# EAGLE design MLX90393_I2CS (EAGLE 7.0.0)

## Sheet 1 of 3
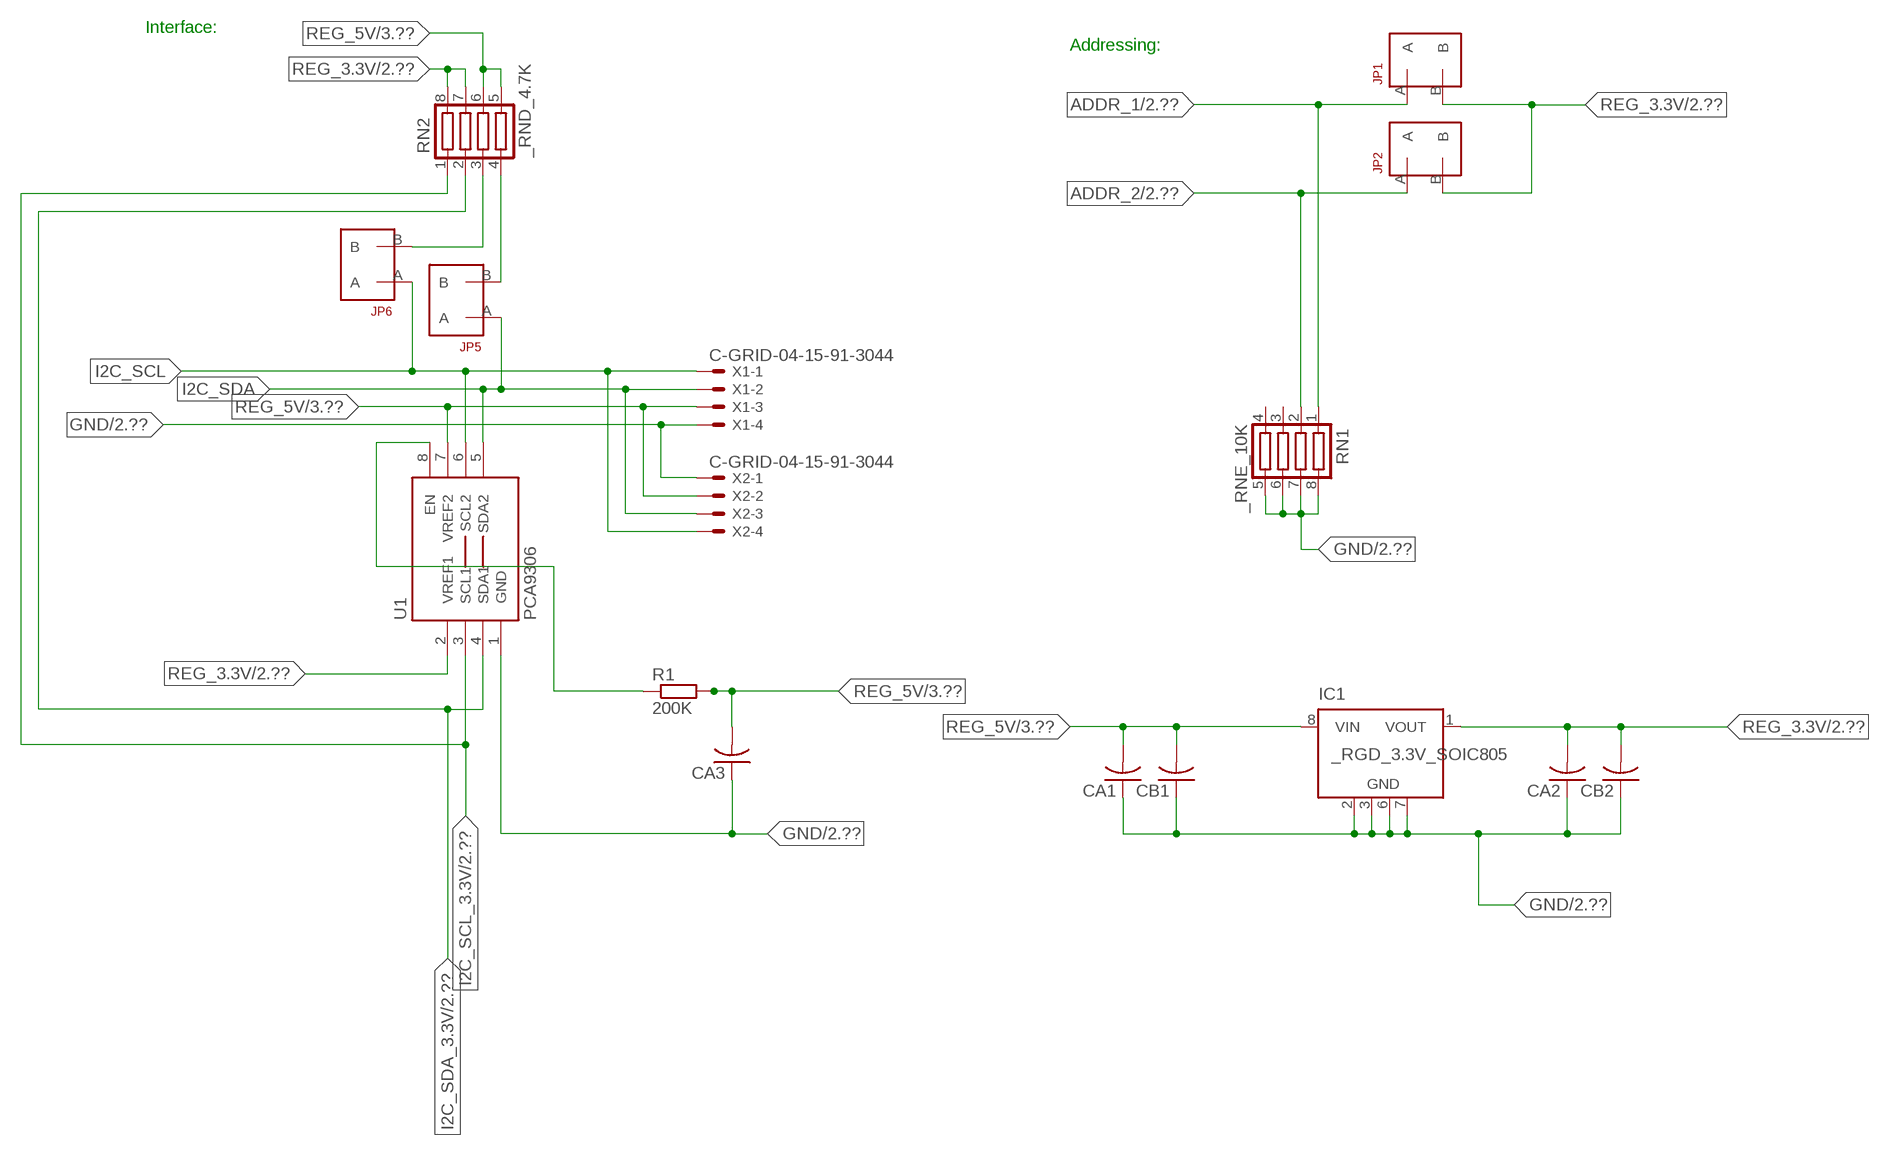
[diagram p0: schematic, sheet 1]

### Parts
CA1  CC1206KRX7R9BB104  [.1UF]
CA2  CC1206KRX7R9BB104  [.1UF]
CA3  CC1206KRX7R9BB104  [.1UF]
CB1  TMK316F106ZL-TC1206K  [TMK316F106ZL-T]
CB2  TMK316F106ZL-TC1206K  [TMK316F106ZL-T]
IC1  _RGD_3.3V_SOIC805  [_RGC_3.3V_SOIC8]
JP1  JUMPER_1X2_2MM  [JUMPER_1X2_2MM]
JP2  JUMPER_1X2_2MM  [JUMPER_1X2_2MM]
JP5  JUMPER_1X2_2MM  [JUMPER_1X2_2MM]
JP6  JUMPER_1X2_2MM  [JUMPER_1X2_2MM]
R1  200K  RESISTOR_SMT-0603  [R603]
RN1  _RNE_10K  [RNE]
RN2  _RND_4.7K  [RND]
U1  PCA9306  PCA9306_NCD  [PSOP-8]
X1  C-GRID-04-15-91-3044  [15-91-04]
X2  C-GRID-04-15-91-3044  [15-91-04]

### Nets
ADDR_1: JP1.A RN1.1 ; also sheet 2
ADDR_2: JP2.A RN1.2 ; also sheet 2
GND: CA1.1 CA2.1 CA3.1 CB1.1 CB2.1 IC1.2(GND) IC1.3(GND) IC1.6(GND) IC1.7(GND) RN1.5 RN1.6 RN1.7 RN1.8 U1.1(GND) X1.4 X2.1 ; also sheet 2,3
I2C_SCL: JP6.A U1.6(SCL2) X1.1 X2.4
I2C_SCL_3.3V: RN2.1 U1.3(SCL1) ; also sheet 2
I2C_SDA: JP5.A U1.5(SDA2) X1.2 X2.3
I2C_SDA_3.3V: RN2.2 U1.4(SDA1) ; also sheet 2
N$1: JP6.B RN2.3
N$2: JP5.B RN2.4
N$3: R1.1 U1.8(EN)
REG_3.3V: CA2.2 CB2.2 IC1.1(VOUT) JP1.B JP2.B RN2.7 RN2.8 U1.2(VREF1) ; also sheet 2
REG_5V: CA1.2 CA3.2 CB1.2 IC1.8(VIN) R1.2 RN2.5 RN2.6 U1.7(VREF2) X1.3 X2.2 ; also sheet 3
Unconnected: IC1.4(NC) IC1.5(NC) RN1.3 RN1.4

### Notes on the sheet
- Interface:
- Addressing:

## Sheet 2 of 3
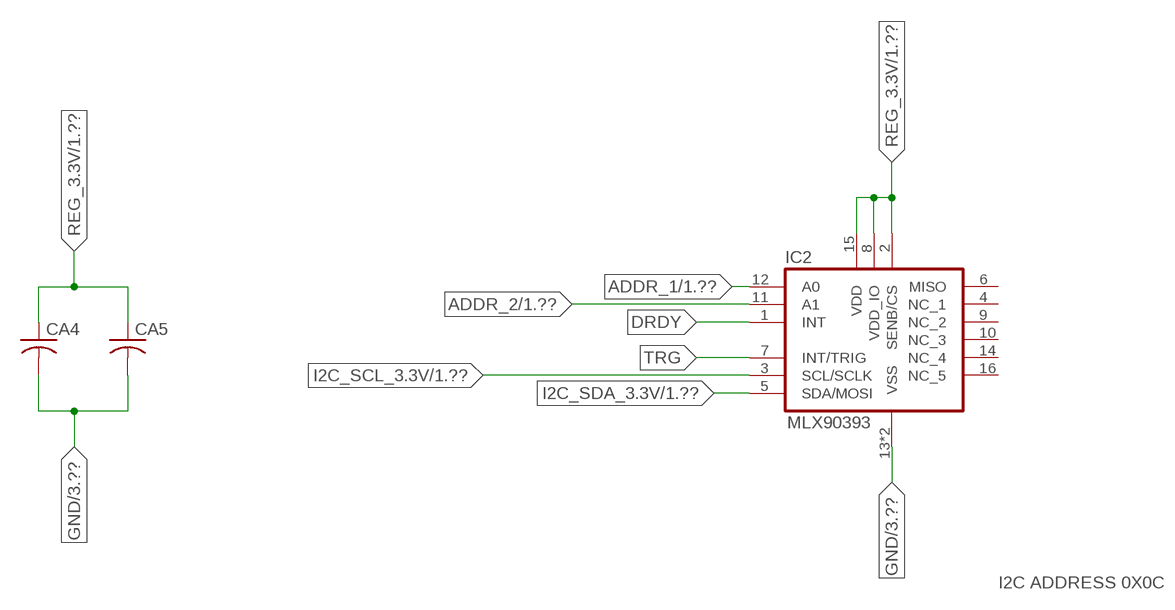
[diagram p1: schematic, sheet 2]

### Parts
CA4  CC1206KRX7R9BB104C1206K  [CC1206KRX7R9BB104]
CA5  CC1206KRX7R9BB104C1206K  [CC1206KRX7R9BB104]
IC2  MLX90393  [MLX90393]

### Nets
ADDR_1: IC2.12(A0) ; also sheet 1
ADDR_2: IC2.11(A1) ; also sheet 1
DRDY: IC2.1(INT)
GND: CA4.2 CA5.2 IC2.13(VSS) IC2.TH(VSS) ; also sheet 1,3
I2C_SCL_3.3V: IC2.3(SCL/SCLK) ; also sheet 1
I2C_SDA_3.3V: IC2.5(SDA/MOSI) ; also sheet 1
REG_3.3V: CA4.1 CA5.1 IC2.2(SENB/CS) IC2.8(VDD_IO) IC2.15(VDD) ; also sheet 1
TRG: IC2.7(INT/TRIG)
Unconnected: IC2.4(NC_1) IC2.6(MISO) IC2.9(NC_2) IC2.10(NC_3) IC2.14(NC_4) IC2.16(NC_5)

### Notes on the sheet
- I2C ADDRESS 0X0C

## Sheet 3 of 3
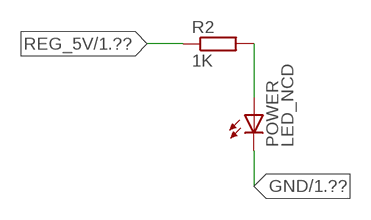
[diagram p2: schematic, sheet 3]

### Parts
POWER  LED_NCD  [CHIPLED_0603]
R2  1K  RESISTOR_SMT-0402  [R402]

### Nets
GND: POWER.C ; also sheet 1,2
N$4: POWER.A R2.2
REG_5V: R2.1 ; also sheet 1

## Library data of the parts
CA1-CA5 = NCD_ULTIMATE_LIBRARY:CC1206KRX7R9BB104: Capacitor CA .1uF 50V SMT C1206K CC1206KRX7R9BB104
CB1 CB2 = NCD_ULTIMATE_LIBRARY:TMK316F106ZL-T: Capacitor CB 10uF SMT 1206 TMK316F106ZL-T
IC1 = NCD_ULTIMATE_LIBRARY:_RGD_3.3V_SOIC8: Regulator Linear 3.3V Chip Positive VOLTAGE REGULATOR Digikey 497-1199-2-ND/L78L33ACD13TR
IC2 = NCD_ULTIMATE_AMAN:MLX90393
JP1 JP2 JP5 JP6 = NCD_ULTIMATE_CONNECTORS:JUMPER_1X2_2MM
POWER = NCD_ULTIMATE_LIBRARY:LED_NCD: LED Digikey 754-1132-2-ND/APT2012SRCPRV
R1 R2 = NCD_ULTIMATE_LIBRARY:RESISTOR_SMT: NCD Resistor
RN1 = NCD_ULTIMATE_LIBRARY:_RNE_10K: Resistor Array RNE SMT 10K x 4 Single Resistor Source: http://www.ctscorp.com/components/Datasheets/CTSChipArrayDs.pdf Digikey 742C083103JPTR-ND/742C083103JP; OC_FARNELL: unknown; OC_NEWARK: unknown
RN2 = NCD_ULTIMATE_LIBRARY:_RND_4.7K: Resistor Array RND SMT 4.7K x 4 Single Resistor Source: http://www.ctscorp.com/components/Datasheets/CTSChipArrayDs.pdf Digikey 742C083472JPTR-ND/742C083472JP; OC_FARNELL: unknown; OC_NEWARK: unknown
U1 = NCD_ULTIMATE_LIBRARY:PCA9306_NCD: NCD Bidirectional I2C level shifter. NOT compatible with all available part number pinout schemes- DOUBLE CHECK!!!; PROD_ID: IC-10023
X1 X2 = NCD_ULTIMATE_CONNECTORS:C-GRID-04: CONNECTOR 4-Pos I2C wire to board 2.54 mm (0.100") pitch header Digikey WM1342-ND/0015912045; OC_FARNELL: unknown; OC_NEWARK: unknown

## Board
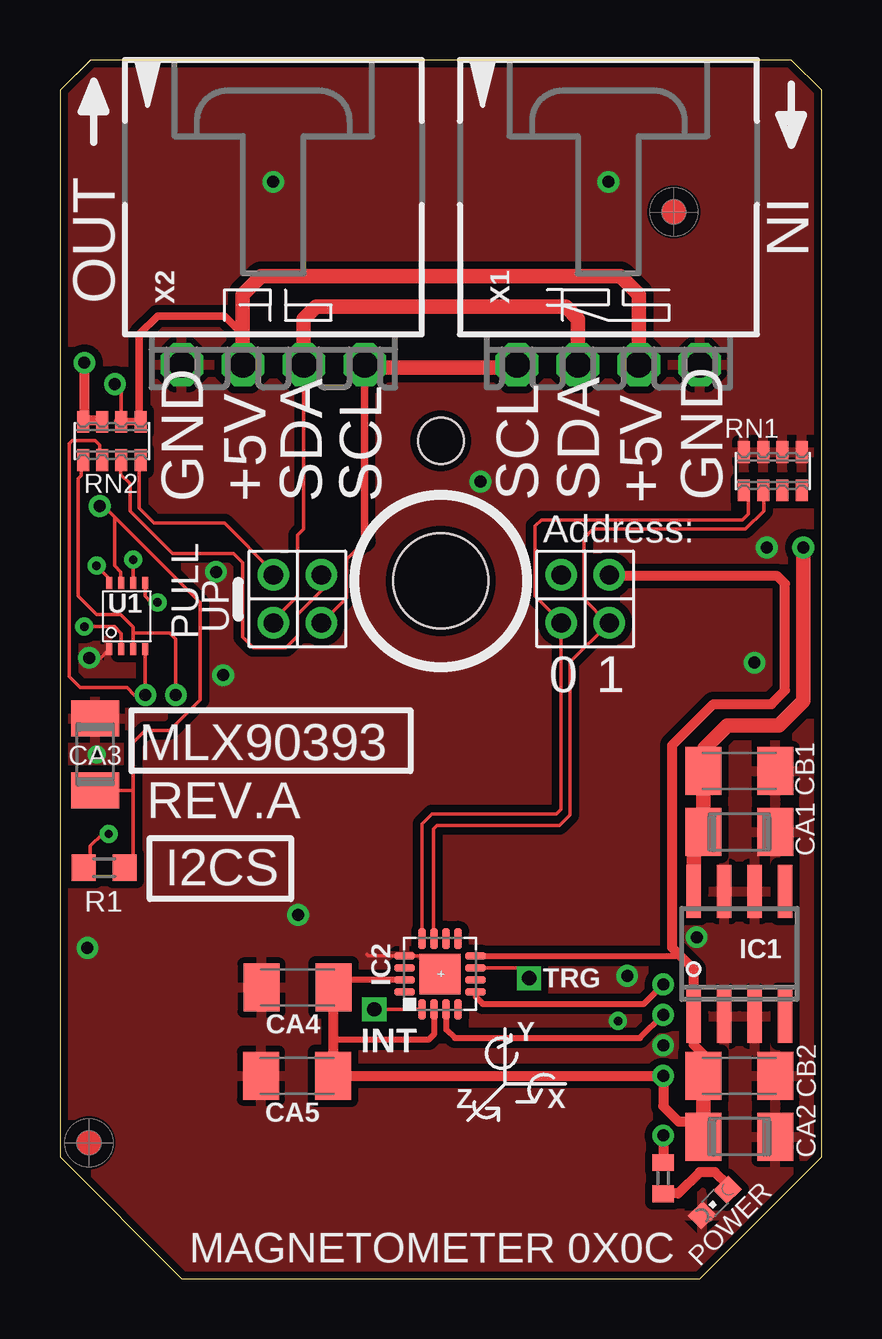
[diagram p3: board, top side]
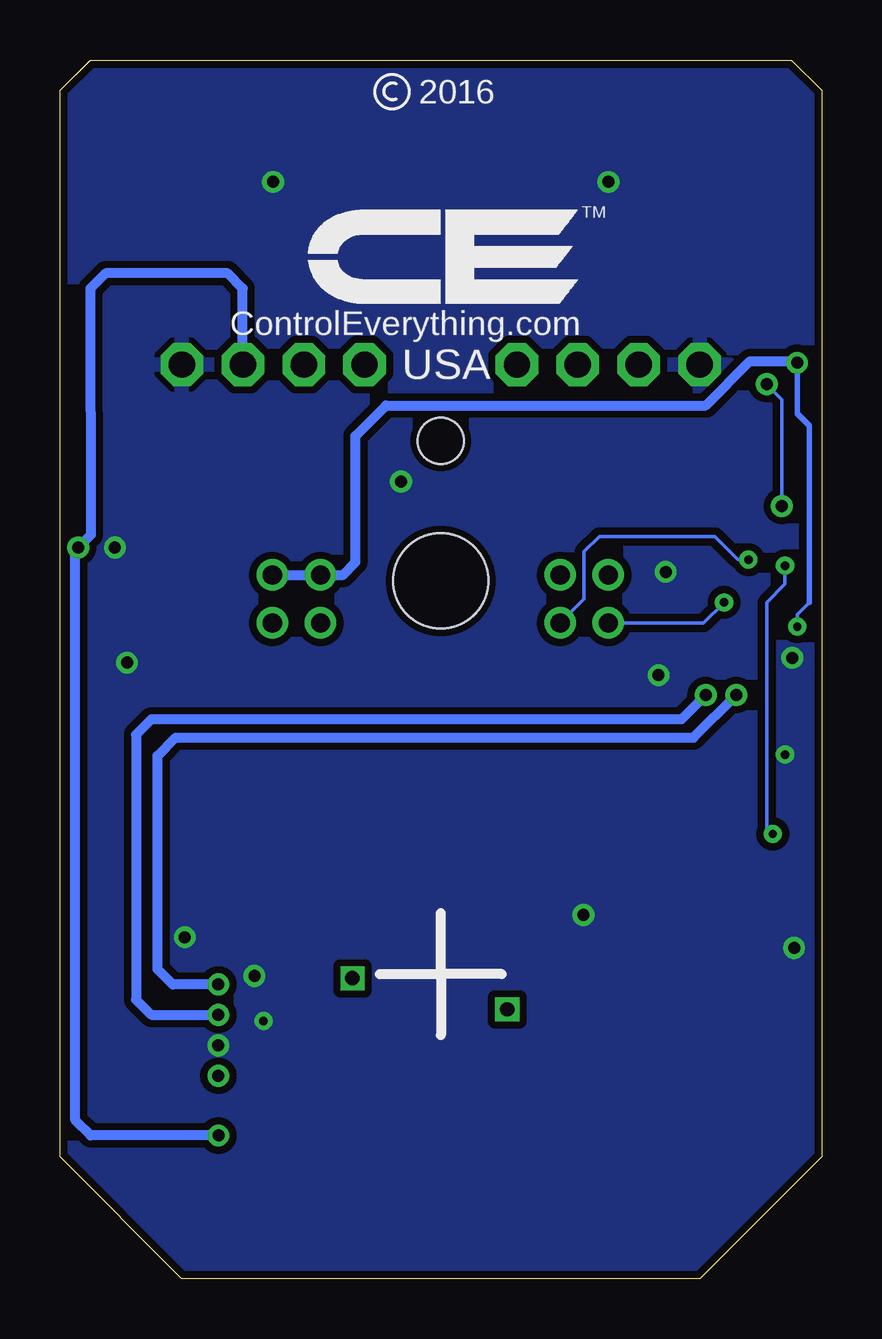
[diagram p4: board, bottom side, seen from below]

Size 31.75 x 50.8 mm. Coordinates in mm from the lower left corner, seen from the top.
Outline: 48 segments
Copper layers (1*16): Top 0.035mm / dielectric 1.5mm / Bottom 0.035mm
Design rules "default": minimum track width 5mil, minimum drill 24mil, track to track 5mil, track to pad 5mil, pad to pad 5mil, via to via 5mil, smd to smd 5mil, copper to edge 10mil, drill to drill 8mil, minimum pad ring 10mil, minimum via ring 8mil, stop-mask expansion 2mil, vias tented up to drill 0mil, thermal gap 10mil
Holes 3.96 mm at 15.88,29.08
Holes 1.91 mm at 15.88,34.93

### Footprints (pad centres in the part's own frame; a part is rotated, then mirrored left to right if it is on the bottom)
.1UF = smd 1.5 x 2: 1 -1.5,0; 2 1.5,0
CC1206KRX7R9BB104 = smd 1.5 x 2: 1 -1.5,0; 2 1.5,0
TMK316F106ZL-T = smd 1.5 x 2: 1 -1.5,0; 2 1.5,0
_RGC_3.3V_SOIC8 = smd 0.6 x 2.2: 1 -1.905,-2.6; 2 -0.635,-2.6; 3 0.635,-2.6; 4 1.905,-2.6; 5 1.905,2.6; 6 0.635,2.6; 7 -0.635,2.6; 8 -1.905,2.6
MLX90393 = smd 0.85 x 0.3: 1 -1.475,0.75; 2 -1.475,0.25; 3 -1.475,-0.25; 4 -1.475,-0.75; 9 1.475,-0.75; 10 1.475,-0.25; 11 1.475,0.25; 12 1.475,0.75 | smd 0.3 x 0.85: 5 -0.75,-1.475; 6 -0.25,-1.475; 7 0.25,-1.475; 8 0.75,-1.475; 13 0.75,1.475; 14 0.25,1.475; 15 -0.25,1.475; 16 -0.75,1.475 | smd 1.7 x 1.7: TH 0,0
JUMPER_1X2_2MM = drill 0.8: A 0,2; B 0,0
CHIPLED_0603 = smd 0.8 x 0.876: A 0,-0.75; C 0,0.75
R603 = smd 1 x 1.1: 1 -0.85,0; 2 0.85,0
R402 = smd 0.7 x 0.9: 1 -0.65,0; 2 0.65,0
RNE = smd 0.5 x 0.9: 1 -1.2,-0.8; 2 -0.4,-0.8; 3 0.4,-0.8; 4 1.2,-0.8; 5 1.2,0.8; 6 0.4,0.8; 7 -0.4,0.8; 8 -1.2,0.8
RND = smd 0.5 x 0.9: 1 -1.2,-0.8; 2 -0.4,-0.8; 3 0.4,-0.8; 4 1.2,-0.8; 5 1.2,0.8; 6 0.4,0.8; 7 -0.4,0.8; 8 -1.2,0.8
PSOP-8 = smd 0.25 x 0.5: 1 -0.73,-1.37; 2 -0.23,-1.37; 3 0.27,-1.37; 4 0.77,-1.37; 5 0.77,1.38; 6 0.27,1.38; 7 -0.23,1.38; 8 -0.73,1.38
15-91-04 = drill 1.1 pad 1.778 octagon: 1 -3.81,-7.62; 2 -1.27,-7.62; 3 1.27,-7.62; 4 3.81,-7.62

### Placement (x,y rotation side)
CA1  28.32,18.62 180 top
CA2  28.32,5.92 180 top
CA3  1.46,21.86 270 top
CA4  9.91,12.14 180 top
CA5  9.88,8.46 180 top
CB1  28.32,21.16 180 top
CB2  28.32,8.46 180 top
IC1  28.32,13.54 0 top
IC2  15.85,12.7 90 top
JP1  20.89,29.34 180 top
JP2  22.9,29.34 180 top
JP5  8.89,29.34 180 top
JP6  10.9,29.34 180 top
POWER  27.3,3.18 135 top
R1  1.84,17.13 0 top
R2  25.15,4.19 270 top
RN1  29.72,33.66 0 top
RN2  2.16,34.93 0 top
U1  2.79,27.61 0 top
U$5  [VISION_REF10]  1.21,5.66 90 top
U$28  [VISION_REF10]  25.59,44.46 90 top
X1  22.86,45.72 0 top
X2  8.89,45.72 0 top

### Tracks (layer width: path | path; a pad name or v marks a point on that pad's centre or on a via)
ADDR_1
  Top 0.152: RN1.1 28.7,32.78 28.7,31.88 28.45,31.62 20.07,31.62 19.81,31.37 19.81,28.45 20.89,27.37 JP1.A 20.88,27.32 20.88,19.56 20.7,19.38 15.52,19.38 15.1,18.96 IC2.12
ADDR_2
  Top 0.152: RN1.2 29.34,32.59 29.34,32 28.57,31.24 22.23,31.24 21.84,30.86 21.84,28.32 22.83,27.34 JP2.A 21.26,25.7 21.26,19.33 20.83,18.9 15.72,18.9 15.57,18.75 15.57,14.5 15.6,14.47 IC2.11
DRDY  (via drill 0.6)
  Top 0.152: IC2.1 v13.11,11.23
GND  (via drill 0.35, 0.5)
  Top 0.152: CA3.1 1.52,23.42 1.52,23.62 | U1.1 1.7,25.88 v1.22,25.88 | IC2.TH 15.1,13.45 IC2.13 12.86,13.45 12.8,13.51
  other vias: 8.89,45.72 22.86,45.72 25.15,9.73 6.8,25.16 17.53,33.22 26.55,14.24 1.15,13.79 6.5,29.46 1.52,21.84 23.65,12.62 23.27,10.74 29.46,30.48 28.96,25.68 9.93,15.16
  pour Top (isolate 0.305): -1.27,0 -1.27,50.8 33.02,50.8 33.02,0
  pour Bottom (isolate 0.305): -5.08,0 -5.08,50.8 35.56,50.8 35.56,0
I2C_SCL  (via drill 0.35)
  Top 0.152: 12.7,30.73 11.94,29.97 11.94,28.38 JP6.A | v3.05,29.97 3.06,29.96 U1.6
  Top 0.305: 12.7,30.73 X2.4
  Top 0.406: X2.4 12.7,37.97 | 19.05,37.97 X1.1
  Top 0.61: 12.7,37.97 19.05,37.97
  Bottom 0.152: JP6.A 9.91,28.33 9.91,30.3 9.27,30.94 4.45,30.94 3.48,29.97 v3.05,29.97
I2C_SCL_3.3V  (via drill 0.5)
  Top 0.152: RN2.1 0.89,34.07 0.89,33.48 0.77,33.35 0.77,29.1 0.76,29.09 0.76,28.45 1.52,27.69 2.54,27.69 3.06,27.17 3.06,26.92 | 3.06,26.92 U1.3 | v4.83,24.33 v4.83,24.34 4.83,26.67 4.57,26.92 3.06,26.92
  Top 0.254: IC2.3 16.1,10.39 16.46,10.03 24.18,10.03 v25.15,11
  Bottom 0.406: v4.83,24.33 5.84,23.32 27.94,23.32 28.58,22.68 28.58,11.63 27.94,11 v25.15,11
I2C_SDA  (via drill 0.35)
  Top 0.152: JP5.A 8.89,27.44 9.91,28.45 9.91,30.99 10.16,31.24 10.16,34.92 X2.3 | U1.5 3.56,28.45 3.81,28.19 v4.06,28.19
  Top 0.61: X2.3 10.16,40.01 10.67,40.51 21.09,40.51 21.59,40.01 X1.2
  Bottom 0.152: v4.06,28.19 4.92,27.34 JP5.A
I2C_SDA_3.3V  (via drill 0.5)
  Top 0.152: RN2.2 1.65,34.14 1.65,34.75 1.46,34.94 0.51,34.94 0.38,34.81 0.38,26.37 0.38,26.36 0.38,25.1 0.84,24.64 2.79,24.64 3.1,24.33 v3.56,24.33 v3.56,24.34 U1.4
  Top 0.254: IC2.5 17.32,11.76 17.63,11.46 24.34,11.46 v25.15,12.27
  Bottom 0.406: v25.15,12.27 27.05,12.27 27.69,12.9 27.69,21.79 26.93,22.56 5.34,22.56 v3.56,24.33
N$1
  Top 0.152: JP6.B 10.92,29.31 10.92,28.7 9.91,27.69 9.91,26.8 9.42,26.31 8.06,26.31 7.62,26.75 7.62,29.84 7.24,30.23 4.7,30.23 2.92,32 2.92,33.15 2.54,33.53 2.54,34.1 RN2.3
  Top 0.305: 2.54,34.02 RN2.3
N$2
  Top 0.152: JP5.B 8.89,29.46 6.86,31.5 3.94,31.5 3.3,32.13 3.3,34.07 RN2.4
  Top 0.305: 3.37,33.88 RN2.4
N$3  (via drill 0.35)
  Top 0.152: R1.1 1.27,17.41 1.27,18.03 1.78,18.54 v2.03,18.54 | v1.52,29.72 2.06,29.18 U1.8
  Bottom 0.152: v2.03,18.54 2.29,18.8 2.29,28.19 1.52,28.96 v1.52,29.72
N$4
  Top 0.406: POWER.A 27.84,3.92 27.3,4.45 26.67,4.45 25.78,3.56 25.16,3.56 R2.2
REG_3.3V  (via drill 0.35, 0.5)
  Top 0.152: v1.02,27.18 2.29,27.18 2.56,26.9 U1.2
  Top 0.254: IC2.15 11.41,12.45 CA4.1 | IC2.8 25.64,13.45 25.76,13.57 | IC2.2 15.6,10.19 15.37,9.96 11.41,9.96 11.41,10.41
  Top 0.406: CB2.2 26.82,9.35 26.42,9.75 26.42,10.36 | 26.82,6.55 25.78,6.55 25.15,7.19 v25.15,8.46 CA5.1 11.41,8.46 11.41,10.41 CA4.1 | IC1.1 26.42,12.9 25.76,13.57 25.53,13.79 25.53,22.24 27.24,23.95 29.66,23.95 30.23,24.52 30.23,28.97 29.91,29.29 22.95,29.29 JP2.B | 26.52,5.62 CA2.2 | v1.02,38.18 1.02,35.78 | 1.02,35.78 RN2.8 | 1.02,35.78 1.71,35.78 RN2.7
  Top 0.61: CB2.2 26.82,6.55 CA2.2 | 26.42,10.36 IC1.1
  Bottom 0.152: 0.51,28.19 1.02,27.69 v1.02,27.18
  Bottom 0.229: 0.51,28.19 0.51,35.56 1.02,36.07 v1.02,38.18
  Bottom 0.406: v1.02,38.18 1.08,38.24 2.99,38.24 4.83,36.4 18.16,36.4 19.43,35.13 19.43,29.87 19.94,29.34 JP1.B JP2.B
REG_5V  (via drill 0.5)
  Top 0.152: RN2.6 2.56,37.01 v2.29,37.29 | R1.2 3.05,17.49 3.05,20.36 | 3.05,20.36 3.05,22.35 3.56,22.86 4.57,22.86 5.84,24.13 5.84,28.19 2.29,31.75 | CA3.2 3.05,20.36 | 2.29,31.75 1.83,32.21 v1.65,32.21 | U1.7 2.54,29.01 2.54,29.46 2.29,29.72 2.29,31.75
  Top 0.305: 7.62,39.37 7.5,39.37 | 2.42,35.74 RN2.6 RN2.5 3.31,35.8 3.31,39.37 4.07,40.13 6.86,40.13 7.62,39.37 | X2.2 7.62,39.37
  Top 0.406: v25.15,5.97 R2.1
  Top 0.61: X1.3 24.13,41.02 23.37,41.78 8.38,41.78 7.62,41.02 X2.2 | IC1.8 26.42,18.21 CA1.2 CB1.2 26.86,21.2 26.86,22.11 27.82,23.06 29.98,23.06 30.99,24.08 v30.99,30.48
  Bottom 0.152: v1.65,32.21 1.65,36.65 v2.29,37.29
  Bottom 0.406: X1.3 24.13,41.28 24.77,41.91 29.84,41.91 30.48,41.27 30.47,31 v30.99,30.48 31.11,30.36 31.11,6.6 30.48,5.97 v25.15,5.97
TRG  (via drill 0.6)
  Top 0.152: IC2.7 19.13,12.95 v19.56,12.52

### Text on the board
tPlace: Y | Z | X
tNames: IN | OUT | GND | +5V | SDA | SCL | SCL | SDA | +5V | GND | Address: | PULL | UP | 0 | 1 | MLX90393 | REV.A | I2CS | TRG | INT | MAGNETOMETER 0X0C
bNames: 2016 | TM | ControlEverything.com | USA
